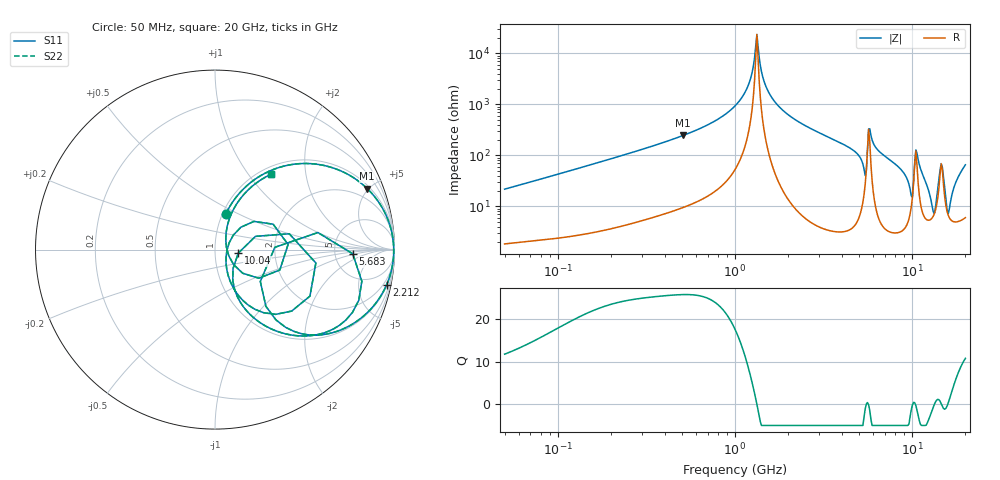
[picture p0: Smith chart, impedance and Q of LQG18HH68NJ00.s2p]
!Murata Part Number: LQG18HH68NJ00
!These Parameters are Measured in Series Mode Connection
!  o--[Z]--o
!Port1  Port2
!  o-------o
!Freq. Start=50[MHz] Stop=20[GHz], 401[Steps]
# Hz S RI R 50
!Freq.(Hz) S11(Real) S11(Imag) S21(Real) S21(Imag) S12(Real) S12(Imag) S22(Real) S22(Imag)
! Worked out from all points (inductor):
!   401 points, 50 MHz to 20 GHz, reference 50 ohm
!   read as one part in series: L = 68.1 nH near 51.52 MHz
!   highest Q = 25.9 at 509.6 MHz (marker M1), where L = 76.5 nH
!   self-resonance near 1.329 GHz
!   S11 on the Smith chart (normalised r, x): 50 MHz: 1.04, +0.43; 2.212 GHz: 1.17, -9.75; 5.683 GHz: 7.51, -0.84; 10.04 GHz: 1.30, -0.05; 20 GHz: 1.12, +1.30
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5e7  0.0602 0.1993  0.9398 -0.1993  0.9398 -0.1993  0.0602 0.1993
1.364002e8  0.2624 0.4167  0.7376 -0.4167  0.7376 -0.4167  0.2624 0.4167
3.721004e8  0.7282 0.4257  0.2718 -0.4257  0.2718 -0.4257  0.7282 0.4257
5.096456e8  0.848 0.3402  0.152 -0.3402  0.152 -0.3402  0.848 0.3402
1e9  0.9828 0.105  0.0172 -0.105  0.0172 -0.105  0.9828 0.105
1.196911e9  0.9937 0.0389  0.0063 -0.0389  0.0063 -0.0389  0.9937 0.0389
1.329223e9  0.9958 4.93e-05  0.00425 -4.93e-05  0.00425 -4.93e-05  0.9958 4.93e-05
1.567309e9  0.9925 -0.0618  0.00754 0.0618  0.00754 0.0618  0.9925 -0.0618
2.211938e9  0.9565 -0.1954  0.0435 0.1954  0.0435 0.1954  0.9565 -0.1954
2.728004e9  0.9096 -0.2797  0.0904 0.2797  0.0904 0.2797  0.9096 -0.2797
4.81993e9  0.5611 -0.4767  0.4389 0.4767  0.4389 0.4767  0.5611 -0.4767
5.352748e9  0.2834 -0.3156  0.7166 0.3156  0.7166 0.3156  0.2834 -0.3156
5.683258e9  0.7671 -0.023  0.2329 0.023  0.2329 0.023  0.7671 -0.023
6.217679e9  0.6652 -0.4392  0.3348 0.4392  0.3348 0.4392  0.6652 -0.4392
7.442007e9  0.4097 -0.473  0.5903 0.473  0.5903 0.473  0.4097 -0.473
9.041845e9  0.1779 -0.343  0.8221 0.343  0.8221 0.343  0.1779 -0.343
1.004137e10  0.13 -0.0194  0.87 0.0194  0.87 0.0194  0.13 -0.0194
1.082228e10  0.4271 -0.3425  0.5729 0.3425  0.5729 0.3425  0.4271 -0.3425
1.334722e10  0.0664 -0.00414  0.9336 0.00414  0.9336 0.00414  0.0664 -0.00414
1.460232e10  0.4072 0.0286  0.5928 -0.0286  0.5928 -0.0286  0.4072 0.0286
1.597544e10  0.0637 0.0134  0.9363 -0.0134  0.9363 -0.0134  0.0637 0.0134
2e10  0.3133 0.42  0.6867 -0.42  0.6867 -0.42  0.3133 0.42
